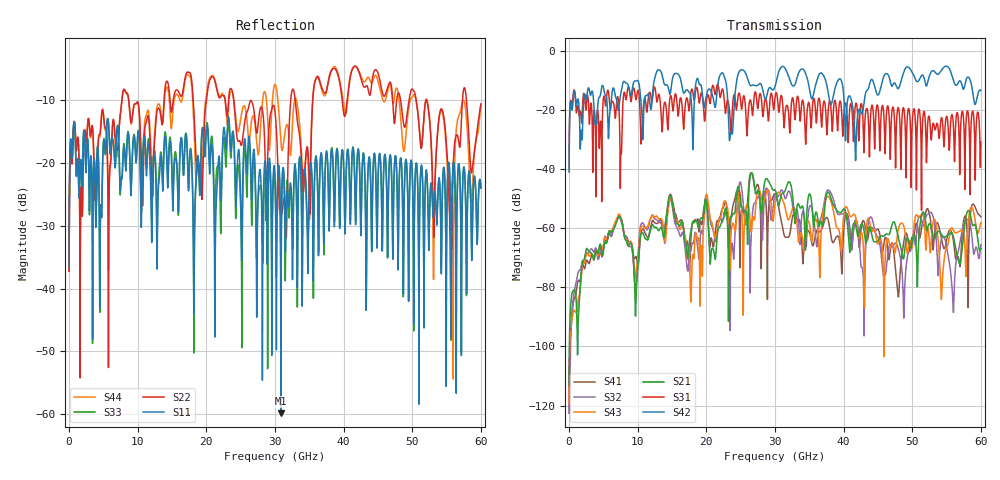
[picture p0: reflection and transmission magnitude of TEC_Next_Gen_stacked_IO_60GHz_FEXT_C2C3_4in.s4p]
!! CHANNEL DESCRIPTION:  Next Generation 28Gbps Press-fit Stacked I/O Connector
!!  with 4" 5-6-5 Megtron 6 Stripline trace on host side and 1.25" 7-5-7 Megtron 6 Microstrip trace on plug side
!! HOST PCB DESCRIPTION:  PCB thickness 3.425 mm
!!  26 Layer Board, 15 GND planes, 4 Layer route-out on Layers 7,11,17,21, 8mil stub on vias
!!  Pairs on following layers
!!  Layer 07 - A02A03 A14A15 D05D06
!!  Layer 11 - D020D3 C05C06 D14D15
!!  Layer 17 - C02C03 B05B06 C14C15
!!  Layer 21 - B02B03 A05A06 B14B15
!! CONNECTOR DESCRIPTION:  Next Generation 28Gbps Press-fit Stacked I/O Connector
!! PLUG-IN CARD DESCRIPTION:  PCB thickness 1mm thick
!!  6 Layer Board, 4 GND planes, 0.35 x 1.4mm mating pads
!!  Micro-strip diff traces referenced to GND plane 3mils down, 2nd GND plane 17mils from top of board
!!  PCB GND planes are symmetric
!! MODEL DESCRIPTION: TE Connectivity S-parameter model produced from Macro-model, Extracted .s4p FEXT (Victim B05B06 - Aggressor C02C03)
!! MODEL DATE: 5/15/2014 CR32f, FPR23
!! MODEL STATUS: Developmental
!! MODEL GEOMETRY: 4 Rows - Rows A, B, C, D. 3 pairs in each row, 12 total pairs
!! MODEL FREQUENCY RANGE: DC to 60 GHz in 10 MHz frequency steps
!! MODEL EDGE RATE LIMITATION: 8.33 ps (Using conservative 0.5/Fmax rule of thumb)
!! TIME-DOMAIN TRANSFORM CAUTIONS:
!! 1.) Do not simulate transient edge rates faster than the number listed above.  Edge
!!  rates faster than this number contain significant spectral content at frequencies
!!  above the model's highest frequency.
!! 2.) Even when simulating edge rates that are slower than the number listed above, be
!!  aware that the best time resolution possible with a direct iFFT is (1 / 2Fmax).
!!  As a result, time resolution is typically not adequate for most time-domain
!!  simulations unless tricks such as frequency-domain zero-padding and windowing are
!!  used to minimize leakage and aliasing.
!! 3.) Because the model has a uniform frequency step, a direct iFFT will result in an
!!  impulse that that has a time length given by either (1 / Fstep) or (1 / 2Fstep),
!!  depending on the transform being used.  Care has been taken in selecting the
!!  frequency step to ensure a settled impulse response for the model.  Therefore,
!!  convolution with the model's impulse response should present no issues.  However,
!!  if directly concatenating s-parameter models in the frequency domain a user must
!!  either interpolate necessary interim frequencies or complete impulse response
!!  zero-padding.  Impulse response zero-padding is more difficult, but more accurate.
!! PORT DEFINITIONS:
!! Port  1  ----->  Host C02		B05 Module <-----  Port  2
!! Port  3  ----->  Host C03		B06 Module <-----  Port  4
! Touchstone data
! Created: 29-Sep-2014 by IdEM R2011 (7.0.3)
# Hz S MA R 50
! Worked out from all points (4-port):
!   6000 points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, 10 MHz to 60 GHz, reference 50 ohm
!   strongest paths, dB at 10 MHz, 15.01 GHz, 30.01 GHz, 45.01 GHz, 60 GHz:
!     S42: -41.0, -10.1, -12.0, -14.9, -13.4
!     S31: -40.0, -17.5, -15.7, -19.1, -30.7
!     S21: -113.2, -51.2, -47.0, -64.2, -66.9
!     S43: -119.2, -51.4, -51.9, -65.3, -58.1
!     S32: -122.6, -52.2, -48.9, -63.0, -65.5
!     S41: -122.5, -50.0, -48.4, -60.3, -56.1
!   lowest |S11| = -59.8 dB at 30.88 GHz (marker M1), VSWR 1.00, Z = 50.1 - j0.0049 ohm
!   |S11| at or under -10 dB: start of sweep to end of sweep
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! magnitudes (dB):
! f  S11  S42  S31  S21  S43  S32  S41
! 10 MHz  -36.5  -41.0  -40.0  -113.2  -119.2  -122.6  -122.5
! 14.75 GHz  -16.6  -14.5  -15.3  -49.0  -50.1  -50.3  -48.5
! 17.38 GHz  -24.2  -13.6  -18.6  -69.2  -68.1  -73.1  -67.0
! 30.88 GHz  -59.8  -5.5  -15.1  -48.9  -49.2  -47.1  -57.1
! 47.92 GHz  -36.0  -12.7  -19.2  -62.7  -60.9  -66.6  -82.4
! 55.58 GHz  -28.1  -6.9  -24.6  -61.6  -60.5  -74.6  -60.7
! 60 GHz  -24.0  -13.4  -30.7  -66.9  -58.1  -65.5  -56.1
